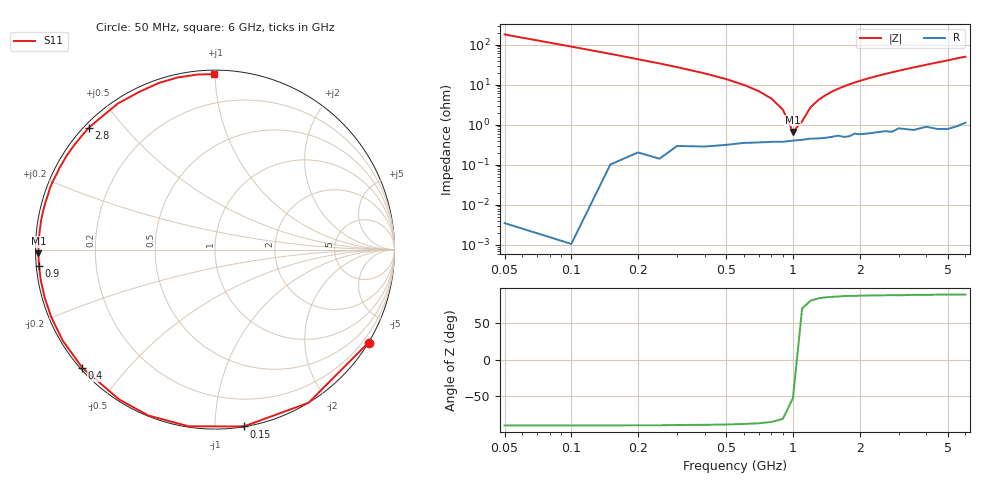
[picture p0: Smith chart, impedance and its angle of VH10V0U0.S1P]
! Infineon Technologies  Discrete & RF Semiconductors
! BB 814
! Si Tuning Diode in SOT23
! VR = 10 V
! S-Parameters:  July  1999
# GHz  S  MA  R  50
!  f  S11
! GHz  MAG  ANG
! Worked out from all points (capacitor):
!   34 points, 50 MHz to 6 GHz, reference 50 ohm
!   read as one part to ground: C = 17.7 pF near 50 MHz
!   lowest |Z| = 658 mohm at 1 GHz (marker M1)
!   series resonance near 1.032 GHz, so ESL is about 1.3 nH
!   S11 on the Smith chart (normalised r, x): 50 MHz: 0.00, -3.58; 150 MHz: 0.00, -1.17; 400 MHz: 0.01, -0.38; 900 MHz: 0.01, -0.05; 2.8 GHz: 0.01, +0.40; 6 GHz: 0.02, +0.99
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0.05  1 -31.2
0.1  1 -58.6
0.15  0.9983 -80.8
0.2  0.9954 -98.5
0.25  0.9961 -111.9
0.3  0.991 -122.6
0.4  0.9901 -138.3
0.5  0.9885 -149.3
0.6  0.9867 -157.7
0.7  0.986 -164.3
0.8  0.9853 -169.8
0.9  0.9852 -174.6
1  0.9842 -178.8
1.1  0.9834 177.4
1.3  0.9822 170.7
1.6  0.9795 162.1
1.8  0.9805 157.0
2  0.9786 152.3
2.2  0.978 147.8
2.4  0.9769 143.7
2.6  0.9762 139.5
2.8  0.9774 135.9
3.5  0.9774 123.6
4  0.975 115.7
4.5  0.9797 108.6
5  0.9812 102.2
5.5  0.9802 95.6
6  0.9777 90.3
